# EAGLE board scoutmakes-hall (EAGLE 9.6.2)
REV: A
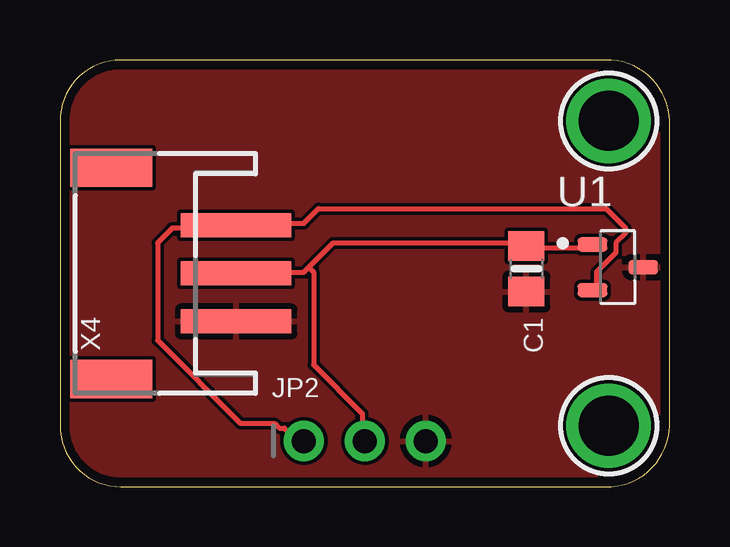
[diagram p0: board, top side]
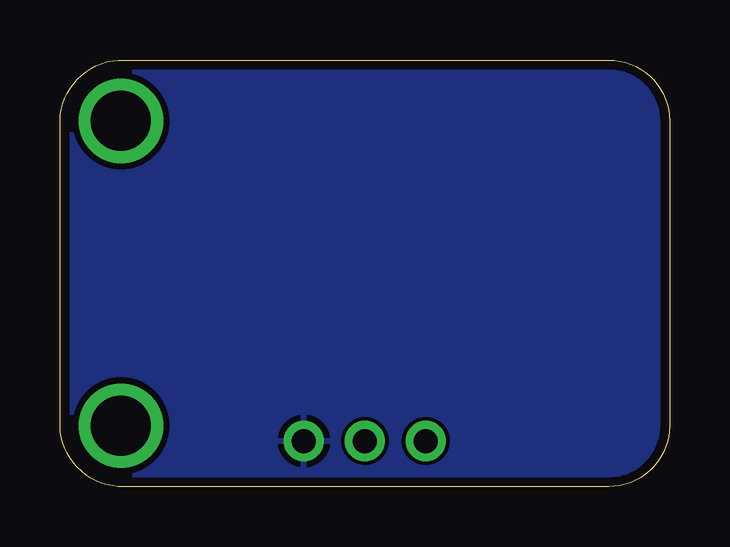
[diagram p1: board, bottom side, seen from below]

Size 25.4 x 17.78 mm. Coordinates in mm from the lower left corner, seen from the top.
Outline: 0,15.24 0,2.54 arc90 2.54,0 22.73,0 arc90 25.4,2.54 25.4,15.24 arc90 22.73,17.78 2.54,17.78 arc90 0,15.24
Copper layers (1*16): Top 0.035559375mm / dielectric 1.6mm / Bottom 0.035559375mm
Design rules "oshpark-2layer *": minimum track width 6mil, minimum drill 10mil, track to track 6mil, track to pad 6mil, pad to pad 6mil, via to via 6mil, smd to smd 6mil, copper to edge 15mil, drill to drill 6mil, minimum pad ring 5mil, minimum via ring 5mil, stop-mask expansion 2.5mil, vias tented up to drill 20mil, thermal gap 10mil
Net classes: 1 HV: width 0.406 mm, drill 0.381 mm, clearance 0.762 mm

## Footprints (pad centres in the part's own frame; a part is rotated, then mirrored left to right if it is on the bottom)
0805-NO = smd 1.24 x 1.5: 1 -0.95,0; 2 0.95,0
1X03_ROUND = drill 1 pad 1.676: 1 -2.54,0; 2 0,0; 3 2.54,0
SOT95P237X112-3N = smd 1.24 x 0.59: 1 -1.055,0.95; 2 -1.055,-0.95; 3 1.055,0
MOUNTINGHOLE_2.5_PLATED = drill 2.5 pad 3.2: P$1 0,0
JSTPH3 = smd 1 x 4.6: 1 -2,-2.7; 2 0,-2.7; 3 2,-2.7 | smd 1.6 x 3.4: NC1 -4.4,2.5; NC2 4.4,2.5

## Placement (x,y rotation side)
C1  10uF  [0805-NO]  19.43,9.08 270 top
JP2  0.1" Header  [1X03_ROUND]  12.7,1.91 0 top
U1  DRV5055A1QDBZT  [SOT95P237X112-3N]  23.24,9.14 0 top
U$1  MOUNTINGHOLE2.5  [MOUNTINGHOLE_2.5_PLATED]  22.86,2.54 0 top
U$8  MOUNTINGHOLE2.5  [MOUNTINGHOLE_2.5_PLATED]  22.86,15.24 0 top
X4  JST PH 3  [JSTPH3]  4.64,8.89 90 top

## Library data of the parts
C1 JP2 = microbuilder
U1 = DRV5055A1QDBZT; AVAILABILITY: In Stock; CHECK_PRICES: https://www.snapeda.com/parts/DRV5055A1QDBZT/Texas+Instruments/view-part/?ref=eda; DESCRIPTION: Ratiometric linear hall effect sensor with analog output; MF: Texas Instruments; MP: DRV5032; PACKAGE: SOT-23-3 Texas Instruments; PRICE: None; PURCHASE-URL: https://www.snapeda.com/api/url_track_click_mouser/?unipart_id=2777465&manufacturer=Texas Instruments&part_name=DRV5055A1QDBZT&search_term=drv5055; SNAPEDA_LINK: https://www.snapeda.com/parts/DRV5055A1QDBZT/Texas+Instruments/view-part/?ref=snap
U$1 U$8 = adafruit_electromech; BOM: EXCLUDE
X4 = adafruit_electromech

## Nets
GND: C1.2 JP2.3 U1.3 X4.1
OUT: JP2.1 U1.2 X4.3
VIN: C1.1 JP2.2 U1.1 X4.2

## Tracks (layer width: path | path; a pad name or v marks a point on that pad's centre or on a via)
GND
  pour Top: 0,17.78 25.4,17.78 25.4,0 0,0
  pour Bottom: 0,17.78 25.4,17.78 25.4,0 0,0
OUT
  Top 0.203: U1.2 22.35,8.33 22.35,8.94 23.16,9.75 23.16,10.16 23.57,10.57 23.57,10.77 22.76,11.58 10.77,11.58 10.16,10.97 7.52,10.97 X4.3 7.32,10.77 4.67,10.77 4.06,10.16 4.06,6.1 7.52,2.64 8.94,2.64 9.14,2.44 9.35,2.44 9.75,2.03 10.16,2.03 JP2.1
VIN
  Top 0.203: U1.1 22.15,9.96 19.51,9.96 C1.1 19.3,10.16 11.38,10.16 10.36,9.14 | 10.36,9.14 10.16,8.94 7.52,8.94 X4.2 | 10.36,9.14 10.57,8.94 10.57,5.08 12.6,3.05 12.6,2.03 JP2.2

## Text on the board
Pinguin_tPlace: OMNIPOLAR / DIGITAL HALL / SENSOR | C1 | U1 | OUT | VIN | GND
Pinguin_bPlace: SCOUTMAKES / HALL EFFECT / SENSOR / DRV5032 | VIN / 1.65V-5.5V | VIN | OUT | GND

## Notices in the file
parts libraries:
microbuilder: This work is placed in the public domain, and may be freely used for commercial and non-commercial work with the following conditions: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
